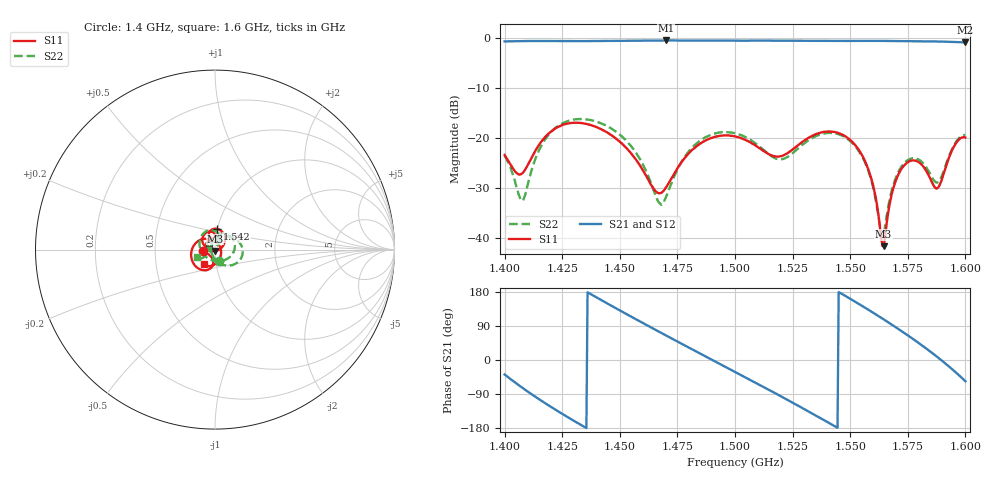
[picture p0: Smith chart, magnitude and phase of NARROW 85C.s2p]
!Agilent Technologies,E8364B,MY43040699,A.07.50.67
!Agilent E8364B: A.07.50.67
!Date: Wednesday, June 25, 2025 06:04:09
!Correction: S11(Full 2 Port(1,2))
!S21(Full 2 Port(1,2))
!S12(Full 2 Port(1,2))
!S22(Full 2 Port(1,2))
!S2P File: Measurements: S11, S21, S12, S22:
# Hz S  dB  R 50
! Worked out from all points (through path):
!   401 points, 1.4 GHz to 1.6 GHz, reference 50 ohm
!   highest |S21| = -0.49 dB at 1.47 GHz (marker M1); lowest = -0.9 dB at 1.6 GHz (marker M2)
!   lowest |S11| = -41.5 dB at 1.565 GHz (marker M3), VSWR 1.02, Z = 49.9 - j0.834 ohm
!   |S11| at or under -10 dB: start of sweep to end of sweep
!   |S22| runs from -39.8 to -16.2 dB; largest |S21 - S12| = 0.00085
!   S11 on the Smith chart (normalised r, x): 1.4 GHz: 0.87, -0.01; 1.542 GHz: 1.00, +0.23; 1.6 GHz: 0.87, -0.14
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1.4e9  -23.35 -173.1  -0.68 -38.2  -0.68 -38.2  -23.47 -68.3
1.4075e9  -27.08 -122.7  -0.61 -72.4  -0.61 -72.4  -32.48 171.9
1.4145e9  -21.63 -97.7  -0.60 -101.7  -0.60 -101.7  -22.83 66.1
1.4245e9  -17.47 -121.1  -0.62 -140.2  -0.62 -140.2  -17.18 19.5
1.4335e9  -16.98 -153.9  -0.62 -172.6  -0.62 -172.6  -16.17 -9.6
1.4425e9  -18.34 170.2  -0.59 156.2  -0.58 156.2  -17.14 -34.5
1.452e9  -21.54 134.1  -0.54 124.2  -0.53 124.2  -20.11 -60.8
1.467e9  -30.99 136.8  -0.49 74.7  -0.49 74.7  -32.85 -157.5
1.47e9  -29.87 154.8  -0.49 64.9  -0.49 64.9  -31.85 148.5
1.4855e9  -20.90 141.8  -0.53 15.1  -0.53 15.1  -20.27 60.3
1.5e9  -19.65 104.5  -0.54 -31.1  -0.54 -31.1  -19.00 8.8
1.517e9  -23.60 97.6  -0.52 -86.1  -0.52 -86.1  -23.91 -89.4
1.5335e9  -19.52 105.3  -0.57 -141.2  -0.57 -141.2  -19.95 146.7
1.542e9  -18.68 84.4  -0.59 -170.2  -0.59 -170.2  -18.95 110.2
1.556e9  -24.15 34.3  -0.57 139.7  -0.58 139.7  -24.40 63.0
1.5645e9  -41.55 -94.2  -0.58 107.3  -0.58 107.4  -39.30 133.0
1.567e9  -33.45 -159.8  -0.59 97.5  -0.59 97.5  -32.50 168.9
1.5705e9  -27.66 173.1  -0.61 83.5  -0.61 83.5  -27.10 169.1
1.5755e9  -24.66 144.6  -0.64 62.9  -0.64 63.0  -24.23 158.1
1.586e9  -29.26 51.1  -0.69 16.6  -0.69 16.6  -28.19 160.3
1.593e9  -23.73 -72.4  -0.76 -17.8  -0.76 -17.8  -23.47 -145.8
1.6e9  -19.88 -128.1  -0.88 -56.0  -0.88 -56.0  -19.39 -155.9
